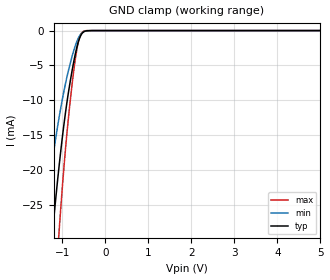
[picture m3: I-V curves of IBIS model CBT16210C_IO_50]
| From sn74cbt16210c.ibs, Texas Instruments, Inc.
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[Model]   CBT16210C_IO_50
Model_type  Terminator
| variable   typ   min   max
C_comp   8.34pF   4.18pF   17.14pF
| C_tri-state   8.34pF   4.18pF   17.14pF
[Temperature Range]   40   100   -40
| Ambient temperature   25   85   -40
[Voltage range]   5   4.5   5.5
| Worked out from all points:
|   GND clamp passes 1 mA (typ) near -0.59 V on its own axis
[GND Clamp]
| CBT16210C_IO
|   Voltage   I(typ)   I(min)   I(max)
-5V       -402.4mA   -301.1mA   -512.1mA
-1.455V   -45.62mA   -29.44mA   -67.39mA
-1.43V    -43.7mA    -28.16mA   -64.65mA
-1.22V    -28.65mA   -18.34mA   -42.75mA
-1.075V   -19.65mA   -12.59mA   -29.15mA
-905mV    -10.99mA   -7.105mA   -15.78mA
-825mV    -7.763mA   -5.016mA   -10.81mA
-735mV    -4.616mA   -2.97mA    -5.968mA
-680mV    -2.974mA   -1.921mA   -3.513mA
-615mV    -1.454mA   -971.3uA   -1.408mA
-495mV    -166.4uA   -143.2uA   -77.2uA
5V        570.8pA    1.883nA    133.3pA
